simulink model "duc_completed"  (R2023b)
settings: Solver=VariableStepAuto  StartTime=0.0  StopTime=100.0  RelTol=1e-3
InitFcn:
  | PreprocIn0data  = dataPreProc('data/input_sig_i0.txt');
  | PreprocIn1data  = dataPreProc('data/input_sig_i1.txt');
  | PreprocOutdata  = dataPreProc('data/output_adder.txt');
undefined symbols (not defined in the file or in its folder): adder, aie, Asymmetric, code, Evaluation, netlist, Platform, S, Symmetric, VCK190, Versal, vsva2197, xcvc1902
libraries: aieDSP x10, matrix_library x6, aieBasic x4, dspsrcs4 x3, aieUtilities x1, vmcUtilities x1

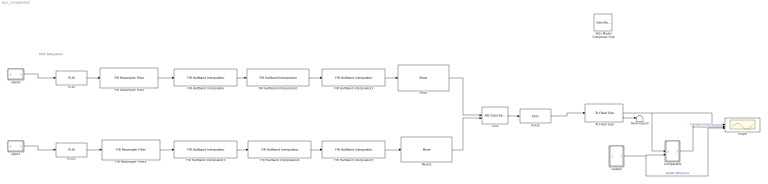
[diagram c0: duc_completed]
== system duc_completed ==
  note: DUC Subsystem
  Comparator : Subsystem
  FIR Halfband Interpolator : aieDSP/FIR Halfband Interpolator  data_type=cint16  coef_type=int16  use_coeff_reload=off  dual_ip=off  num_outputs=off  coeff=[90, -522, 1814, -5208, 20212, 32767]  fir_length=31  input_window_size=384  shift_val=15  rnd_mode=Round symmetrical to infinity  sat_mode=3-Symmetric  interp_poly=1  upshift_ct=0  casc_length=1  AIE_VARIANT=1  blockJsonConstraints=[]  blockJsonConstraintsInternal=[]  spec=vmc_fir_interpolate_hb.json  SerializedMaskParamNames=[]  SerializedMaskParamValues=[]  SerializedMaskParamVisibilities=[]  block_type=FIR Halfband Interpolator  SerializedMaskParamDataypes=typename|typename|bool|bool|bool|coef_type|uint|uint|uint|uint|uint|uint|uint|uint|uint  SerializedMaskParamEnumStrArr=0|0|0|0|0|0|0|0|0|Floor,Ceiling,Round to positive infinity,Round to negative infinity,Round symmetrical to infinity,Round symmetrical to zero,Round convergent to even,Round convergent to odd|0-None,1-Asymmetric,3-Symmetric|0|0|0|0  SerializedMaskParamEnumValArr=0|0|0|0|0|0|0|0|0|0,1,2,3,4,5,6,7|0,1,3|0|0|0|0  SerializedMaskParamVectorArr=0|0|0|0|0|1|0|0|0|0|0|0|0|0|0
  FIR Halfband Interpolator1 : aieDSP/FIR Halfband Interpolator  data_type=cint16  coef_type=int16  use_coeff_reload=off  dual_ip=off  num_outputs=off  coeff=[479, -3461, 19366, 32767]  fir_length=31  input_window_size=768  shift_val=15  rnd_mode=Round symmetrical to infinity  sat_mode=3-Symmetric  interp_poly=1  upshift_ct=0  casc_length=1  AIE_VARIANT=1  blockJsonConstraints=[]  blockJsonConstraintsInternal=[]  spec=vmc_fir_interpolate_hb.json  SerializedMaskParamNames=[]  SerializedMaskParamValues=[]  SerializedMaskParamVisibilities=[]  block_type=FIR Halfband Interpolator  SerializedMaskParamDataypes=typename|typename|bool|bool|bool|coef_type|uint|uint|uint|uint|uint|uint|uint|uint|uint  SerializedMaskParamEnumStrArr=0|0|0|0|0|0|0|0|0|Floor,Ceiling,Round to positive infinity,Round to negative infinity,Round symmetrical to infinity,Round symmetrical to zero,Round convergent to even,Round convergent to odd|0-None,1-Asymmetric,3-Symmetric|0|0|0|0  SerializedMaskParamEnumValArr=0|0|0|0|0|0|0|0|0|0,1,2,3,4,5,6,7|0,1,3|0|0|0|0  SerializedMaskParamVectorArr=0|0|0|0|0|1|0|0|0|0|0|0|0|0|0
  FIR Halfband Interpolator2 : aieDSP/FIR Halfband Interpolator  data_type=cint16  coef_type=int16  use_coeff_reload=off  dual_ip=off  num_outputs=off  coeff=[-2117, 18499, 32767]  fir_length=31  input_window_size=1536  shift_val=15  rnd_mode=Round symmetrical to infinity  sat_mode=3-Symmetric  interp_poly=1  upshift_ct=0  casc_length=1  AIE_VARIANT=1  blockJsonConstraints=[]  blockJsonConstraintsInternal=[]  spec=vmc_fir_interpolate_hb.json  SerializedMaskParamNames=[]  SerializedMaskParamValues=[]  SerializedMaskParamVisibilities=[]  block_type=FIR Halfband Interpolator  SerializedMaskParamDataypes=typename|typename|bool|bool|bool|coef_type|uint|uint|uint|uint|uint|uint|uint|uint|uint  SerializedMaskParamEnumStrArr=0|0|0|0|0|0|0|0|0|Floor,Ceiling,Round to positive infinity,Round to negative infinity,Round symmetrical to infinity,Round symmetrical to zero,Round convergent to even,Round convergent to odd|0-None,1-Asymmetric,3-Symmetric|0|0|0|0  SerializedMaskParamEnumValArr=0|0|0|0|0|0|0|0|0|0,1,2,3,4,5,6,7|0,1,3|0|0|0|0  SerializedMaskParamVectorArr=0|0|0|0|0|1|0|0|0|0|0|0|0|0|0
  FIR Halfband Interpolator3 : aieDSP/FIR Halfband Interpolator  data_type=cint16  coef_type=int16  use_coeff_reload=off  dual_ip=off  num_outputs=off  coeff=[90, -522, 1814, -5208, 20212, 32767]  fir_length=31  input_window_size=384  shift_val=15  rnd_mode=Round symmetrical to infinity  sat_mode=3-Symmetric  interp_poly=1  upshift_ct=0  casc_length=1  AIE_VARIANT=1  blockJsonConstraints=[]  blockJsonConstraintsInternal=[]  spec=vmc_fir_interpolate_hb.json  SerializedMaskParamNames=[]  SerializedMaskParamValues=[]  SerializedMaskParamVisibilities=[]  block_type=FIR Halfband Interpolator  SerializedMaskParamDataypes=typename|typename|bool|bool|bool|coef_type|uint|uint|uint|uint|uint|uint|uint|uint|uint  SerializedMaskParamEnumStrArr=0|0|0|0|0|0|0|0|0|Floor,Ceiling,Round to positive infinity,Round to negative infinity,Round symmetrical to infinity,Round symmetrical to zero,Round convergent to even,Round convergent to odd|0-None,1-Asymmetric,3-Symmetric|0|0|0|0  SerializedMaskParamEnumValArr=0|0|0|0|0|0|0|0|0|0,1,2,3,4,5,6,7|0,1,3|0|0|0|0  SerializedMaskParamVectorArr=0|0|0|0|0|1|0|0|0|0|0|0|0|0|0
  FIR Halfband Interpolator4 : aieDSP/FIR Halfband Interpolator  data_type=cint16  coef_type=int16  use_coeff_reload=off  dual_ip=off  num_outputs=off  coeff=[479, -3461, 19366, 32767]  fir_length=31  input_window_size=768  shift_val=15  rnd_mode=Round symmetrical to infinity  sat_mode=3-Symmetric  interp_poly=1  upshift_ct=0  casc_length=1  AIE_VARIANT=1  blockJsonConstraints=[]  blockJsonConstraintsInternal=[]  spec=vmc_fir_interpolate_hb.json  SerializedMaskParamNames=[]  SerializedMaskParamValues=[]  SerializedMaskParamVisibilities=[]  block_type=FIR Halfband Interpolator  SerializedMaskParamDataypes=typename|typename|bool|bool|bool|coef_type|uint|uint|uint|uint|uint|uint|uint|uint|uint  SerializedMaskParamEnumStrArr=0|0|0|0|0|0|0|0|0|Floor,Ceiling,Round to positive infinity,Round to negative infinity,Round symmetrical to infinity,Round symmetrical to zero,Round convergent to even,Round convergent to odd|0-None,1-Asymmetric,3-Symmetric|0|0|0|0  SerializedMaskParamEnumValArr=0|0|0|0|0|0|0|0|0|0,1,2,3,4,5,6,7|0,1,3|0|0|0|0  SerializedMaskParamVectorArr=0|0|0|0|0|1|0|0|0|0|0|0|0|0|0
  FIR Halfband Interpolator5 : aieDSP/FIR Halfband Interpolator  data_type=cint16  coef_type=int16  use_coeff_reload=off  dual_ip=off  num_outputs=off  coeff=[-2117, 18499, 32767]  fir_length=31  input_window_size=1536  shift_val=15  rnd_mode=Round symmetrical to infinity  sat_mode=3-Symmetric  interp_poly=1  upshift_ct=0  casc_length=1  AIE_VARIANT=1  blockJsonConstraints=[]  blockJsonConstraintsInternal=[]  spec=vmc_fir_interpolate_hb.json  SerializedMaskParamNames=[]  SerializedMaskParamValues=[]  SerializedMaskParamVisibilities=[]  block_type=FIR Halfband Interpolator  SerializedMaskParamDataypes=typename|typename|bool|bool|bool|coef_type|uint|uint|uint|uint|uint|uint|uint|uint|uint  SerializedMaskParamEnumStrArr=0|0|0|0|0|0|0|0|0|Floor,Ceiling,Round to positive infinity,Round to negative infinity,Round symmetrical to infinity,Round symmetrical to zero,Round convergent to even,Round convergent to odd|0-None,1-Asymmetric,3-Symmetric|0|0|0|0  SerializedMaskParamEnumValArr=0|0|0|0|0|0|0|0|0|0,1,2,3,4,5,6,7|0,1,3|0|0|0|0  SerializedMaskParamVectorArr=0|0|0|0|0|1|0|0|0|0|0|0|0|0|0
  FIR Resampler Filter : aieDSP/FIR Resampler Filter  data_type=cint16  coef_type=int16  use_coeff_reload=off  num_outputs=off  coeff=[-8,-15,2,27,38,-1,-67,-86,1,139,171,-2,-257,-309,2,443,522,-3,-724,-842,4,1144,1324,-4,-1789,-2078,5,2866,3402,-5,-5080,-6495,6,13412,27026,32762,27026,13412,6,-6495,-5080,-5,3402,2866,5,-2078,-1789,-4,1324,1144,4,-842,-724,-3,522,443,2,-309,-257,-2,171,139,1,-86,-67,-1,38,27,2,-15,-8]  fir_length=30  interpolate_factor=3  decimate_factor=2  input_window_size=256  shift_val=15  rnd_mode=Round symmetrical to infinity  sat_mode=3-Symmetric  interp_poly=1  deci_poly=1  casc_length=1  AIE_VARIANT=1  blockJsonConstraints=[]  blockJsonConstraintsInternal=[]  spec=vmc_fir_resampler.json  SerializedMaskParamNames=[]  SerializedMaskParamValues=[]  SerializedMaskParamVisibilities=[]  block_type=FIR Resampler Filter  SerializedMaskParamDataypes=typename|typename|bool|bool|coef_type|uint|uint|uint|uint|uint|uint|uint|uint|uint|uint|uint  SerializedMaskParamEnumStrArr=0|0|0|0|0|0|0|0|0|0|Floor,Ceiling,Round to positive infinity,Round to negative infinity,Round symmetrical to infinity,Round symmetrical to zero,Round convergent to even,Round convergent to odd|0-None,1-Asymmetric,3-Symmetric|0|0|0|0  SerializedMaskParamEnumValArr=0|0|0|0|0|0|0|0|0|0|0,1,2,3,4,5,6,7|0,1,3|0|0|0|0  SerializedMaskParamVectorArr=0|0|0|0|1|0|0|0|0|0|0|0|0|0|0|0
  FIR Resampler Filter1 : aieDSP/FIR Resampler Filter  data_type=cint16  coef_type=int16  use_coeff_reload=off  num_outputs=off  coeff=[-8,-15,2,27,38,-1,-67,-86,1,139,171,-2,-257,-309,2,443,522,-3,-724,-842,4,1144,1324,-4,-1789,-2078,5,2866,3402,-5,-5080,-6495,6,13412,27026,32762,27026,13412,6,-6495,-5080,-5,3402,2866,5,-2078,-1789,-4,1324,1144,4,-842,-724,-3,522,443,2,-309,-257,-2,171,139,1,-86,-67,-1,38,27,2,-15,-8]  fir_length=30  interpolate_factor=3  decimate_factor=2  input_window_size=256  shift_val=15  rnd_mode=Round symmetrical to infinity  sat_mode=3-Symmetric  interp_poly=1  deci_poly=1  casc_length=1  AIE_VARIANT=1  blockJsonConstraints=[]  blockJsonConstraintsInternal=[]  spec=vmc_fir_resampler.json  SerializedMaskParamNames=[]  SerializedMaskParamValues=[]  SerializedMaskParamVisibilities=[]  block_type=FIR Resampler Filter  SerializedMaskParamDataypes=typename|typename|bool|bool|coef_type|uint|uint|uint|uint|uint|uint|uint|uint|uint|uint|uint  SerializedMaskParamEnumStrArr=0|0|0|0|0|0|0|0|0|0|Floor,Ceiling,Round to positive infinity,Round to negative infinity,Round symmetrical to infinity,Round symmetrical to zero,Round convergent to even,Round convergent to odd|0-None,1-Asymmetric,3-Symmetric|0|0|0|0  SerializedMaskParamEnumValArr=0|0|0|0|0|0|0|0|0|0|0,1,2,3,4,5,6,7|0,1,3|0|0|0|0  SerializedMaskParamVectorArr=0|0|0|0|1|0|0|0|0|0|0|0|0|0|0|0
  Golden : Subsystem
  Mixer : aieDSP/Mixer  data_type=cint16  input_window_size=3072  rnd_mode=Round symmetrical to infinity  sat_mode=1-Asymmetric  mixer_mode=Single Input Mode  USE_PHASE_RELOAD=off  phase_increment=715827883  AIE_VARIANT=1  blockJsonConstraints=[]  blockJsonConstraintsInternal=[]  spec=vmc_mixer.json  SerializedMaskParamNames=[]  SerializedMaskParamValues=[]  SerializedMaskParamVisibilities=[]  block_type=Mixer  SerializedMaskParamDataypes=typename|uint|uint|uint|uint|bool|uint|uint  SerializedMaskParamEnumStrArr=0|0|Floor,Ceiling,Round to positive infinity,Round to negative infinity,Round symmetrical to infinity,Round symmetrical to zero,Round convergent to even,Round convergent to odd|0-None,1-Asymmetric,3-Symmetric|Single Input Mode,Dual Input Mode|0|0|0  SerializedMaskParamEnumValArr=0|0|0,1,2,3,4,5,6,7|0,1,3|1,2|0|0|0  SerializedMaskParamVectorArr=0|0|0|0|0|0|0|0
  Mixer1 : aieDSP/Mixer  data_type=cint16  input_window_size=3072  rnd_mode=Round symmetrical to infinity  sat_mode=1-Asymmetric  mixer_mode=Single Input Mode  USE_PHASE_RELOAD=off  phase_increment=3042268501  AIE_VARIANT=1  blockJsonConstraints=[]  blockJsonConstraintsInternal=[]  spec=vmc_mixer.json  SerializedMaskParamNames=[]  SerializedMaskParamValues=[]  SerializedMaskParamVisibilities=[]  block_type=Mixer  SerializedMaskParamDataypes=typename|uint|uint|uint|uint|bool|uint|uint  SerializedMaskParamEnumStrArr=0|0|Floor,Ceiling,Round to positive infinity,Round to negative infinity,Round symmetrical to infinity,Round symmetrical to zero,Round convergent to even,Round convergent to odd|0-None,1-Asymmetric,3-Symmetric|Single Input Mode,Dual Input Mode|0|0|0  SerializedMaskParamEnumValArr=0|0|0,1,2,3,4,5,6,7|0,1,3|1,2|0|0|0  SerializedMaskParamVectorArr=0|0|0|0|0|0|0|0
  PLIO : aieBasic/PLIO  PlioWidth=64  PlioFreqSpec=off  PlioFreq=250  ColLocation=0  channel=0  blockJsonConstraints=[]  deprecateConstraints=0
  PLIO1 : aieBasic/PLIO  PlioWidth=64  PlioFreqSpec=off  PlioFreq=250  ColLocation=0  channel=0  blockJsonConstraints=[]  deprecateConstraints=0
  PLIO2 : aieBasic/PLIO  PlioWidth=64  PlioFreqSpec=off  PlioFreq=250  ColLocation=0  channel=0  blockJsonConstraints=[]  deprecateConstraints=0
  Scope : Scope  NumInputPorts=3
  Terminator2 : Terminator
  To Fixed Size : aieUtilities/To Fixed Size  Mode=Produce a valid output signal  OutputSize=3072  CopyMethod=Buffer samples to form output  HasStatusOutput=on
  Vitis Model Composer Hub : vmcUtilities/Vitis Model Composer Hub  Tag=genX  CodeGeneration=off  SubsystemName=DUC Subsystem  CompilationType=AIECompilation  ExportTypeV2=Graph Code  TargetDirectory=./code  exportDesign=off  analyzeDesign=on  validateDesignOnHw=off  ExportType=AI Engines  IpVendor=xilinx.com  IpLibrary=hls  IpVersion=1.0  IpHWLanguage=Verilog  AieCompilerOptions={}  AieSimulatorOptions={}  CreateTestbench=on  TestbenchStackSize=10  RunRtlSim=off  RunCSim=off  RunAieSim=on  AieSimTimeout=50000  RunAieSimProfiling=off  LaunchVitisAnalyzer=off  PlotOutput=off  RunX86Sim=off  X86SimTimeout=10  GenHwImage=off  GenLibadfXo=off  GenHwValidationCode=off  PlatformType=Not Specified  HwSystemType=Baremetal  HwValidationTarget=hw  ProjDevice=Versal VCK190 Evaluation Platform (xcvc1902-vsva2197-2MP-e-S)  ProjDevicePart=xcvc1902-vsva2197-2MP-e-S  AIEType=AIE  SamplePeriod=-1  ClockFrequency=200  DataPathParallelism=1  xilinxfamily=versalaicore  part=xcvc1902  speed=-2MP-e-S  package=vsva2197  directory=./netlist  testbench=off  incr_netlist=off  synthesis_tool=Vivado  clock_wrapper=Clock Enables  dbl_ovrd=According to Block Masks  dcm_input_clock_period=10  sysclk_period=10  simulink_period=1  eval_field=0  IPInfoJsonString="{\"AIESubsystem\":{\"SubsystemName\":\"DUC_Subsystem\",\"TargetDirectory\":\"./code\",\"SubsystemDir\":\"./code/ip/DUC_Subsystem\"},\"SubsystemTag\":\"AIENode\"}"  LogFileName=/home/amd/training/vmc_test/lab/code/model_composer.log  NThreads=4
  input0 : Subsystem
  input1 : Subsystem
  run1 : aieBasic/AIE Class Kernel  KernelAllAttrs=s[12;12;9;9;19;14;21;23;21;23;24;21;15;17;12;24;26;26;26;27;28;9;21;23;23;23;24;25;14;19;19;29]@FunctionNameDeclFileNamePortNamesPortTypesPortSerializedTypesPortDirectionsPortWindowSizeEnablesPortWindowMarginEnablesPortBufferSizeEnablesPortBufferMarginEnablesPortSynchronicityEnablesPortSignalSizeEnablesPortBufferSizesPortBufferMarginsFunctionDeclFunctionTemplateSpecKindFunctionTemplateParamNamesFu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  PortNames={'mixer_i0'; 'mixer_i1'; 'y'}  PortSerializedTypes={'{Q2{R{Tadf::input_buffer{2{t{Scint16}}{t{Tadf::extents{1{t{}3072}}}}}}}}'; '{Q2{R{Tadf::input_buffer{2{t{Scint16}}{t{Tadf::extents{1{t{}3072}}}}}}}}'; '{Q2{R{Tadf::output_buffer{2{t{Scint16}}{t{Tadf::extents{1{t{}3072}}}}}}}}'}  PortWindowSizes={3.072000000000000000e+03; 3.072000000000000000e+03; 3.072000000000000000e+03}  PortWindowMargins={0.000000000000000000e+00; 0.000000000000000000e+00; 0.000000000000000000e+00}  PortSynchronicities={'sync', 'sync', 'sync'}  PortSignalSizes={0.000000000000000000e+00; 0.000000000000000000e+00; 0.000000000000000000e+00}  ClassTemplateSpecKind=none  ClassTemplateParamNames={}  ClassTemplateParamKinds={}  ClassTemplateParamTypes={}  ClassTemplateParamValues={}  ClassCtorParamNames={}  ClassCtorParamSerializedTypes={}  ClassCtorParamValues={}  ClassIndex=1  ClassCtorIndex=0  ClassTabVisible=on  ClassTemplateParamsVisible=off  ClassCtorDeclVisible=off  ClassCtorParamsVisible=off  FunctionTabVisible=on  FunctionDecl=|  PortAttrs={ 'input', 'mixer_i0', 'adf::input_buffer< cint16, adf::extents< 3072 > > & restrict', '3072', '0', 'sync', ''; 'input', 'mixer_i1', 'adf::input_buffer< cint16, adf::extents< 3072 > > & restrict', '3072', '0', 'sync', ''; 'output', 'y', 'adf::output_buffer< cint16, adf::extents< 3072 > > & restrict', '3072', '', 'sync', '' }  PortAttrsEnables={'off', 'off', 'off', 'off', 'off', 'off', 'off';'off', 'off', 'off', 'off', 'off', 'off', 'off';'off', 'off', 'off', 'off', 'off', 'off', 'off'}  SampleTime=-1  ClassDeclTypeOptions=C[1 1]@t12@class adder;  ClassDecl=class adder;  ClassTemplateParams={}  ClassTemplateParamsEnables={}  ClassCtorDeclTypeOptions=C[1 1]@t7@<empty>  ClassCtorDecl=<empty>  ClassCtorParams={}  KernelHeaderFile=aie/adder.h  KernelClassName=adder  KernelFunction=run  KernelSourceFile=aie/adder.cpp  KernelSearchPaths={}  PreProcOptions={}  blockJsonConstraints=[]
      | void adder::
      | run(adf::input_buffer< cint16, adf::extents< 3072 > > & restrict mixer_i0, adf::input_buffer< cint16, adf::extents< 3072 > > & restrict mixer_i1, adf::output_buffer< cint16, adf::extents< 3072 > > & restrict y)
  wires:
  To Fixed Size/1 -> Scope/1, Comparator/1(In1)
  To Fixed Size/2 -> Terminator2/1
  Golden/1(Out1) -> Scope/3, Comparator/2(In2)  "Golden Reference"
  Comparator/1(Out1) -> Scope/2  "Compare Output"
  PLIO2/1 -> To Fixed Size/1
  PLIO/1 -> FIR Resampler Filter/1
  FIR Halfband Interpolator4/1 -> FIR Halfband Interpolator5/1
  Mixer/1 -> run1/1
  input0/1(Out1) -> PLIO/1
  FIR Resampler Filter1/1 -> FIR Halfband Interpolator3/1
  FIR Halfband Interpolator3/1 -> FIR Halfband Interpolator4/1
  FIR Halfband Interpolator2/1 -> Mixer/1
  FIR Halfband Interpolator1/1 -> FIR Halfband Interpolator2/1
  FIR Halfband Interpolator/1 -> FIR Halfband Interpolator1/1
  input1/1(Out1) -> PLIO1/1
  run1/1 -> PLIO2/1
  FIR Resampler Filter/1 -> FIR Halfband Interpolator/1
  FIR Halfband Interpolator5/1 -> Mixer1/1
  Mixer1/1 -> run1/2
  PLIO1/1 -> FIR Resampler Filter1/1

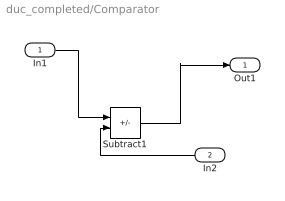
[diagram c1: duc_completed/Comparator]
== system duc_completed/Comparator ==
  In1 : Inport
  In2 : Inport  Port=2
  Subtract1 : Sum  Inputs=+-  OutDataTypeStr=double
  Out1 : Outport
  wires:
  In1/1 -> Subtract1/1
  In2/1 -> Subtract1/2
  Subtract1/1 -> Out1/1

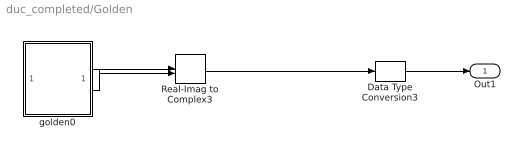
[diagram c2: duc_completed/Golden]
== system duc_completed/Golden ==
  Data Type Conversion3 : DataTypeConversion  OutDataTypeStr=int16
  Real-Imag to Complex3 : RealImagToComplex
  golden0 : Subsystem
  Out1 : Outport
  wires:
  Real-Imag to Complex3/1 -> Data Type Conversion3/1
  golden0/2(Out2) -> Real-Imag to Complex3/2
  golden0/1(Out1) -> Real-Imag to Complex3/1
  Data Type Conversion3/1 -> Out1/1

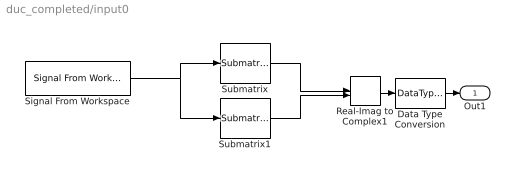
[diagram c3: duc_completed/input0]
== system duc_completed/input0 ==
  Data Type Conversion : DataTypeConversion  OutDataTypeStr=int16
  Real-Imag to Complex1 : RealImagToComplex
  Signal From Workspace : dspsrcs4/Signal From Workspace  X=PreprocIn0data  Ts=1  nsamps=256  OutputAfterFinalValue=Setting to zero  ignoreOrWarnInputAndFrameLengths=off  OutputFrames=off
  Submatrix : matrix_library/Submatrix  RowSpan=All rows  RowStartMode=First  RowStartIndex=1  RowEndMode=Last  RowEndIndex=1  ColSpan=One column  ColStartMode=First  ColStartIndex=1  ColEndMode=Last  ColEndIndex=1
  Submatrix1 : matrix_library/Submatrix  RowSpan=All rows  RowStartMode=First  RowStartIndex=1  RowEndMode=Last  RowEndIndex=1  ColSpan=One column  ColStartMode=Last  ColStartIndex=1  ColEndMode=Last  ColEndIndex=1
  Out1 : Outport
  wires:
  Signal From Workspace/1 -> Submatrix1/1, Submatrix/1
  Submatrix/1 -> Real-Imag to Complex1/1
  Submatrix1/1 -> Real-Imag to Complex1/2
  Real-Imag to Complex1/1 -> Data Type Conversion/1
  Data Type Conversion/1 -> Out1/1

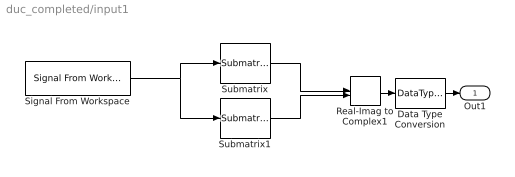
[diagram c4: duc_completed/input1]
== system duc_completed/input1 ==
  Data Type Conversion : DataTypeConversion  OutDataTypeStr=int16
  Real-Imag to Complex1 : RealImagToComplex
  Signal From Workspace : dspsrcs4/Signal From Workspace  X=PreprocIn1data  Ts=1  nsamps=256  OutputAfterFinalValue=Setting to zero  ignoreOrWarnInputAndFrameLengths=off  OutputFrames=off
  Submatrix : matrix_library/Submatrix  RowSpan=All rows  RowStartMode=First  RowStartIndex=1  RowEndMode=Last  RowEndIndex=1  ColSpan=One column  ColStartMode=First  ColStartIndex=1  ColEndMode=Last  ColEndIndex=1
  Submatrix1 : matrix_library/Submatrix  RowSpan=All rows  RowStartMode=First  RowStartIndex=1  RowEndMode=Last  RowEndIndex=1  ColSpan=One column  ColStartMode=Last  ColStartIndex=1  ColEndMode=Last  ColEndIndex=1
  Out1 : Outport
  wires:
  Signal From Workspace/1 -> Submatrix1/1, Submatrix/1
  Submatrix/1 -> Real-Imag to Complex1/1
  Submatrix1/1 -> Real-Imag to Complex1/2
  Real-Imag to Complex1/1 -> Data Type Conversion/1
  Data Type Conversion/1 -> Out1/1

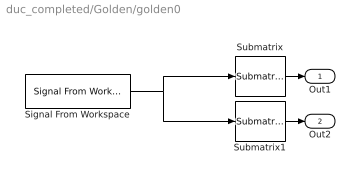
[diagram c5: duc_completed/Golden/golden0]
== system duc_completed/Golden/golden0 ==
  Signal From Workspace : dspsrcs4/Signal From Workspace  X=PreprocOutdata  Ts=1  nsamps=3072  OutputAfterFinalValue=Setting to zero  ignoreOrWarnInputAndFrameLengths=on  OutputFrames=off
  Submatrix : matrix_library/Submatrix  RowSpan=All rows  RowStartMode=First  RowStartIndex=1  RowEndMode=Last  RowEndIndex=1  ColSpan=One column  ColStartMode=First  ColStartIndex=1  ColEndMode=Last  ColEndIndex=1
  Submatrix1 : matrix_library/Submatrix  RowSpan=All rows  RowStartMode=First  RowStartIndex=1  RowEndMode=Last  RowEndIndex=1  ColSpan=One column  ColStartMode=Last  ColStartIndex=1  ColEndMode=Last  ColEndIndex=1
  Out1 : Outport  VectorParamsAs1DForOutWhenUnconnected=off
  Out2 : Outport  Port=2  VectorParamsAs1DForOutWhenUnconnected=off
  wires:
  Submatrix/1 -> Out1/1
  Signal From Workspace/1 -> Submatrix/1, Submatrix1/1
  Submatrix1/1 -> Out2/1
